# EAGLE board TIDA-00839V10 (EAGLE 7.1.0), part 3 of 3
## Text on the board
tPlace: 50 mA MAX | 50 mA MAX | 50 mA MAX | 50 mA MAX | 120/240 Vrms | 120/240 Vrms | 120/240 Vrms | 50/60 Hz | 50/60 Hz | 50/60 Hz
tNames: VCC | DGND | RTCCLK | RS232 | ACT | DGND | DGND | REACT | REACT | ACT | GND | ISOLATED | REACTIVE | + | + | + | + | + | + | + | + | M. MESGANAW / OCTOBER 2015 | RS232_GND | RS232_VCC | DVCC | INTERNAL | EXTERNAL | TIDA-00839 | J=JTAG | J | S | S=SBW | Version 1.0 | For more designs, visit www.ti.com/smartgrid | DVCC | VCC_PL | VCC_ISO | AUXVCC1 | AUXVCC2 | AUXVCC3 | DGND | DGND | VDSYS | VOLTAGE | CURRENT | Danger | Danger | High Voltage | High Voltage
_tplace: RS1 | C80 | TX_EN | VCC | DVCC | DGND | RTCCLK | C79 | * | RX_EN | C77 | * | RS232 | DGND | ACT | U5 | U8 | U6 | DGND | DGND | REACT | C76 | C78 | 5 | REACT | ACT | RTC | GND | 9 | C72 | 4 | C75 | ISOLATED | 8 | * | ISO_PULSE | C73 | REACTIVE | 3 | C74 | LED3 | LED2 | LED1 | LED_ACT | LED_REACT | LED4 | LED5 | LED6 | 7 | C71 | 2 | * | 6 | ABTN4 | DBTN1 | 1 | C70 | D51 | R54 | + | R55 | + | R56 | + | R57 | + | R58 | + | R59 | + | R60 | + | R61 | + | U7 | M. MESGANAW / OCTOBER 2015 | D50 | C69 | RS232_GND | RS232_VCC | R52 | R53 | DVCC | 1 | 2 | INTERNAL | ABTN3 | DBTN2 | EXTERNAL | RESET | TIDA-00839 | 14 | LCD1 | R49 | R50 | R51 | R48 | C53 | J=JTAG | J | S | S=SBW | JTAG | Version 1.0 | For more designs, visit www.ti.com/smartgrid | D23 | DVCC | R46 | C58 | R4 | C36 | C47 | D26 | R43 | * | R95 | C61 | C60 | C49 | R35 | U3 | R98 | R42 | D18 | C48 | D19 | D20 | D21 | D22 | R97 | 1 | DRVPWR4 | R37 | C45 | R38 | VCC_PL | VCC_ISO | R96 | D27 | JP3 | MSP430F67791A | C62 | D17 | R39 | C43 | C44 | C40 | T1 | DRV-I1 | D46 | C38 | XT1 | C34 | U4 | C35 | U$6 | C37 | R104 | 1 | C66 | C30 | C33 | R92 | U4GND | C31 | C32 | R93 | R94 | C50 | C22 | C23 | C29 | C28 | C39 | C46 | C52 | U6GND | 1 | U6OUT | C24 | C25 | C26 | C27 | AUXVCC1 | AUXVCC2 | AUXVCC3 | 1 | U5OUT | R45 | 1 | 1 | 1 | C56 | 1 | R68 | U$5 | D25 | R62 | U$4 | D24 | U$8 | 1 | R36 | DGND | DGND | VDSYS | R65 | 1 | 1 | U5GND | U4OUT | 1 | DRVPWR1 | C63 | DRV-I | VOLTAGE | CURRENT | C14 | C15 | C16 | C17 | C18 | C19 | C20 | C21 | C8 | C9 | R32 | C10 | C11 | R33 | C12 | C13 | R34 | R24 | R25 | R26 | R27 | R28 | R29 | R30 | R31 | R20 | C4 | R21 | C5 | R22 | C6 | R23 | C7 | C1 | R14 | R15 | C2 | R16 | R17 | C3 | R18 | R19 | R/L7 | R/L8 | R/L9 | R/L10 | R/L12 | R/L14 | R/L11 | TVS1 | TVS2 | TVS3 | R/L13 | TVS4 | D9 | D10 | D11 | D12 | D13 | D14 | D15 | D16 | R10 | R7 | R13 | D41 | D43 | D29 | D31 | D33 | D35 | D37 | D39 | R6 | R9 | R12 | R8 | R5 | R11 | L6 | D40 | D42 | D28 | D30 | D32 | D34 | D36 | D38 | Danger | Danger | L3 | L1 | High Voltage | High Voltage | L5 | D1 | D2 | D3 | D4 | D5 | D6 | D7 | D8 | R1 | R2 | R3 | IN+ | IN- | I1+ | I1- | I2+ | I2- | I3+ | I3- | 50 mA MAX | 50 mA MAX | 50 mA MAX | 50 mA MAX | LINE1 | LINE2 | LINE3 | 120/240 Vrms | 120/240 Vrms | 120/240 Vrms | 50/60 Hz | 50/60 Hz | 50/60 Hz | NEUTRAL | C51 | 1 | R44 | 1 | U3GND | C41 | 1 | C42 | 1 | R40 | 1 | U1GND | U2GND | R41 | 1 | C57 | R67 | U$3 | U$1 | 1 | U$2 | U$7 | U3OUT | 1 | 1 | U1OUT | 1 | U2OUT
_bplace: L7 | C102 | R66 | C67 | C68 | D49 | R108 | D47 | R107 | C55 | R64 | R105 | C64 | R106 | D48 | R47 | C65 | R63 | C54 | D45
